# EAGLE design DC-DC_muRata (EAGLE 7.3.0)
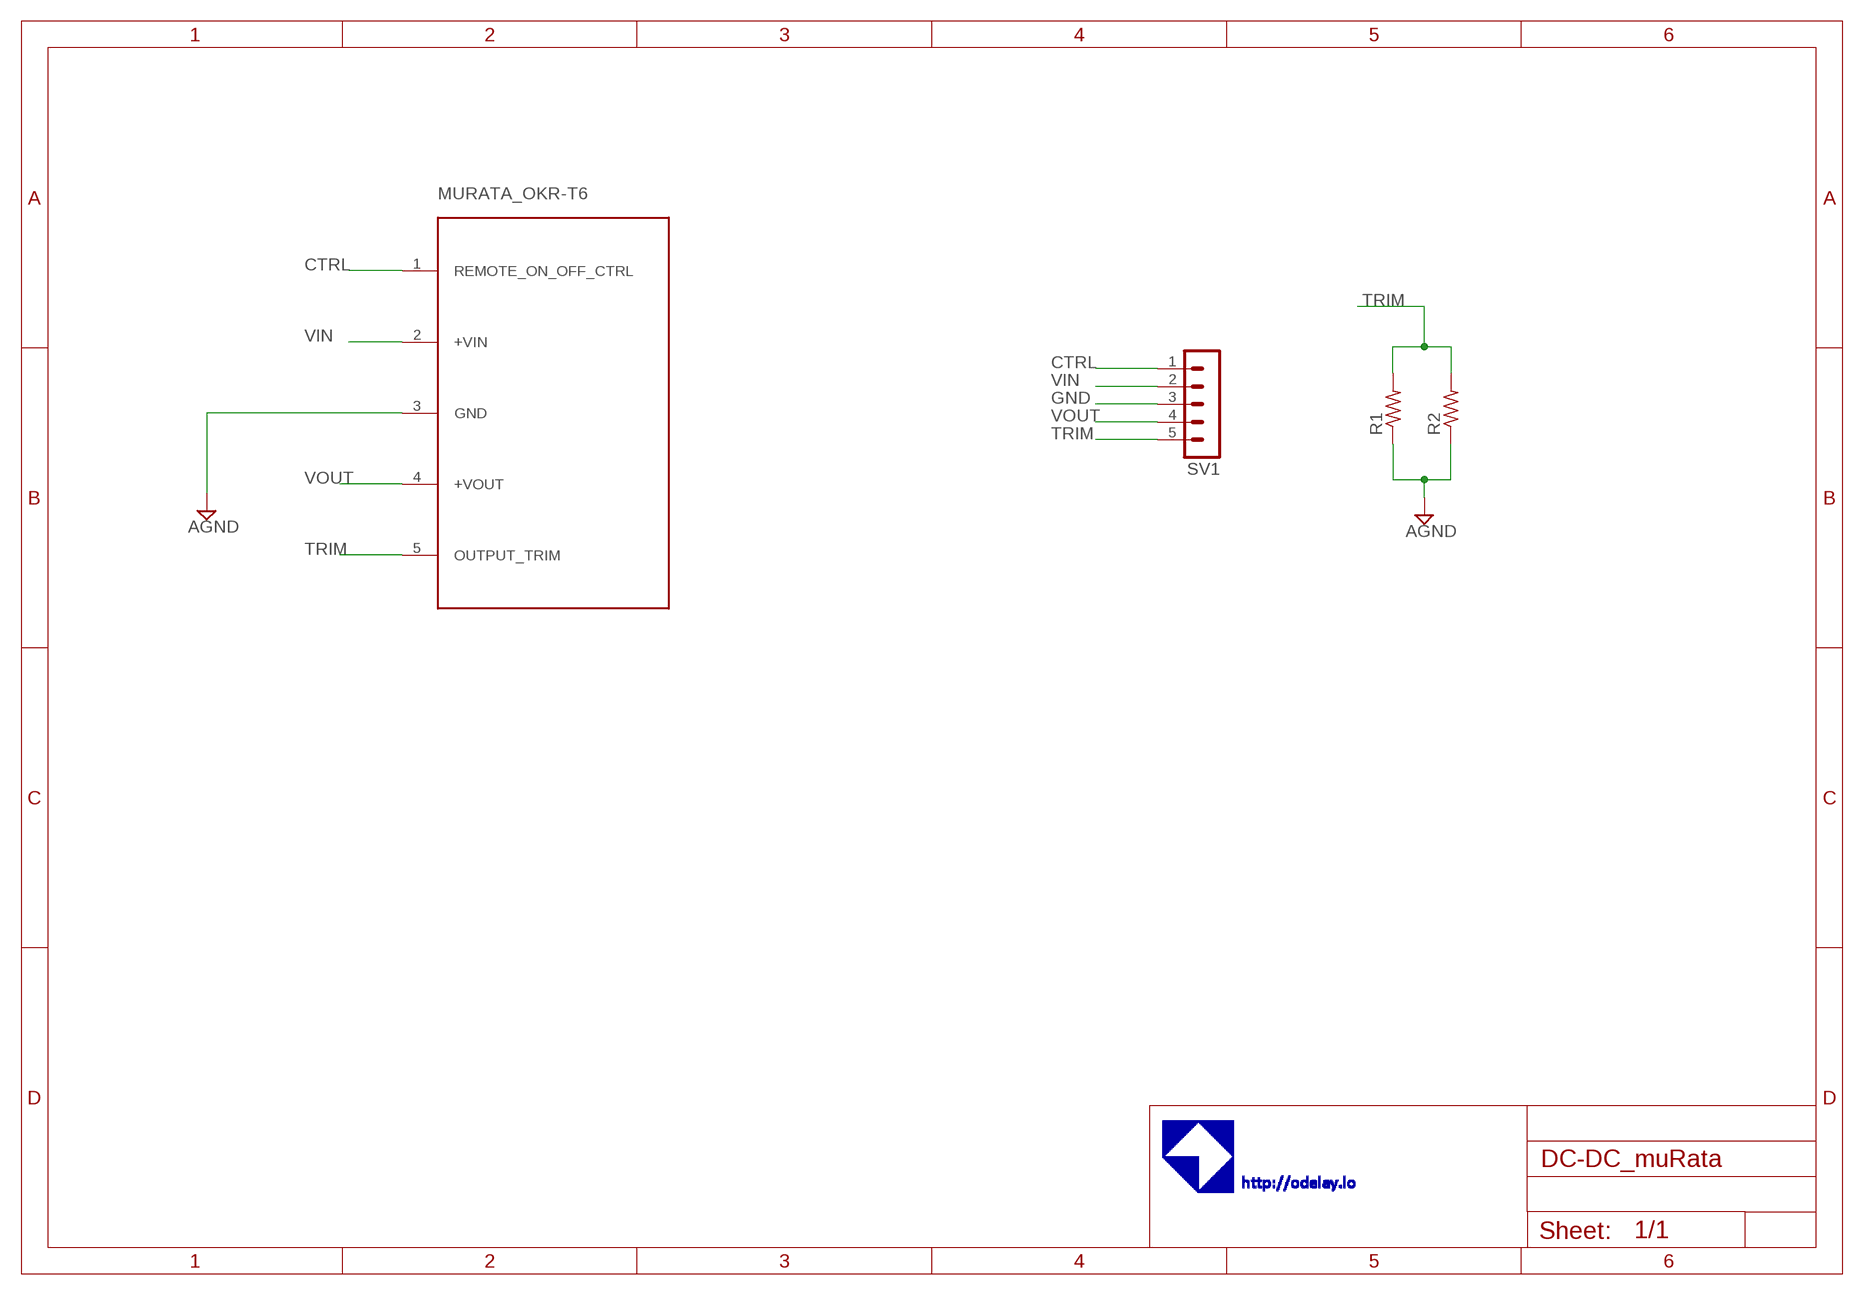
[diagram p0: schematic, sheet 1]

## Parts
MURATA_OKR-T6  MURATA_OKR_T6_DC-DCSIP-5-DCDC  [SIP-5-OKR]
R1  R-US_R0805  [R0805]
R2  R-US_0204/7  [0204/7]
SV1  MA05-1  [MA05-1]

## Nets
CTRL: MURATA_OKR-T6.1(REMOTE_ON_OFF_CTRL) SV1.1
GND: MURATA_OKR-T6.3(GND) R1.1 R2.1 SV1.3 ; supply symbol labelled AGND
TRIM: MURATA_OKR-T6.5(OUTPUT_TRIM) R1.2 R2.2 SV1.5
VIN: MURATA_OKR-T6.2(+VIN) SV1.2
VOUT: MURATA_OKR-T6.4(+VOUT) SV1.4

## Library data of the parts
MURATA_OKR-T6 = odelay:MURATA_OKR_T6_DC-DC
R1 R2 = resistor:R-US_: RESISTOR, American symbol
SV1 = con-lstb:MA05-1: PIN HEADER; OC_FARNELL: unknown; OC_NEWARK: unknown

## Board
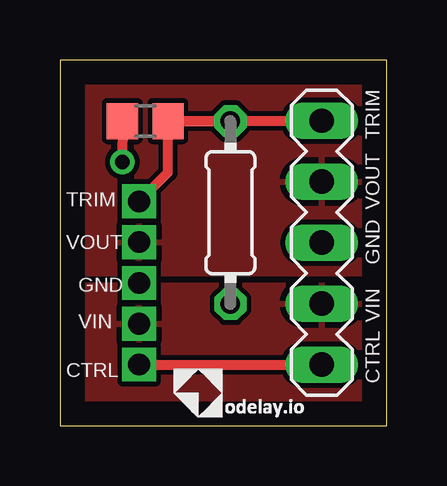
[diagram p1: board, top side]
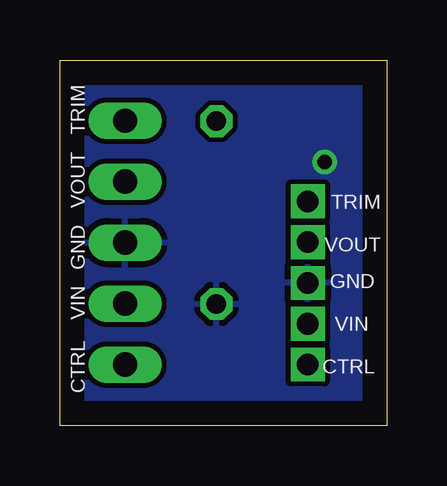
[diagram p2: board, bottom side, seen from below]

Size 13.64 x 15.23 mm. Coordinates in mm from the lower left corner, seen from the top.
Outline: 0,0 13.64,0 13.64,15.23 0,15.23 0,0
Copper layers (1*16): Top 0.035mm / dielectric 1.5mm / Bottom 0.035mm
Design rules "default": minimum track width 10mil, minimum drill 24mil, track to track 8mil, track to pad 8mil, pad to pad 8mil, via to via 8mil, smd to smd 8mil, copper to edge 40mil, drill to drill 8mil, minimum pad ring 10mil, minimum via ring 8mil, stop-mask expansion 4mil, vias tented up to drill 0mil, thermal gap 10mil

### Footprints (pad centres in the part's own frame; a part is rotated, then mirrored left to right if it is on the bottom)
SIP-5-OKR = drill 0.9 square: 1 0,0; 2 1.7,0; 3 3.4,0; 4 5.1,0; 5 6.8,0
R0805 = smd 1.3 x 1.5: 1 -0.95,0; 2 0.95,0
0204/7 = drill 0.813 octagon: 1 -3.81,0; 2 3.81,0
MA05-1 = drill 1.016 long: 1 -5.08,0; 2 -2.54,0; 3 0,0; 4 2.54,0; 5 5.08,0

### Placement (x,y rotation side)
MURATA_OKR-T6  3.3,2.54 90 top
R1  3.56,12.68 0 top
R2  7.11,8.87 90 top
SV1  10.92,7.62 90 top

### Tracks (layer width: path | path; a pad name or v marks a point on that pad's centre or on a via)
CTRL
  Top 0.406: MURATA_OKR-T6.1 SV1.1
GND  (via drill 0.61)
  Top 0.406: R1.1 v2.6,10.98
  pour Bottom: 0.51,14.71 13.21,14.71 13.21,0.49 0.51,0.49
TRIM
  Top 0.406: MURATA_OKR-T6.5 4.51,10.54 R1.2 | R1.2 R2.2 | R1.2 4.53,12.7 SV1.5
VIN
  pour Top: 0.51,5.82 0.51,0.74 12.95,0.74 12.95,5.82
VOUT
  pour Top: 0.51,14.71 12.95,14.71 12.95,6.33 0.51,6.33

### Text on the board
tPlace: TRIM | TRIM | VOUT | VOUT | GND | GND | VIN | VIN | CTRL | CTRL
bPlace: TRIM | VOUT | TRIM | VOUT | GND | GND | VIN | VIN | CTRL | CTRL
Measures: Diameter Drill = 0.9mm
